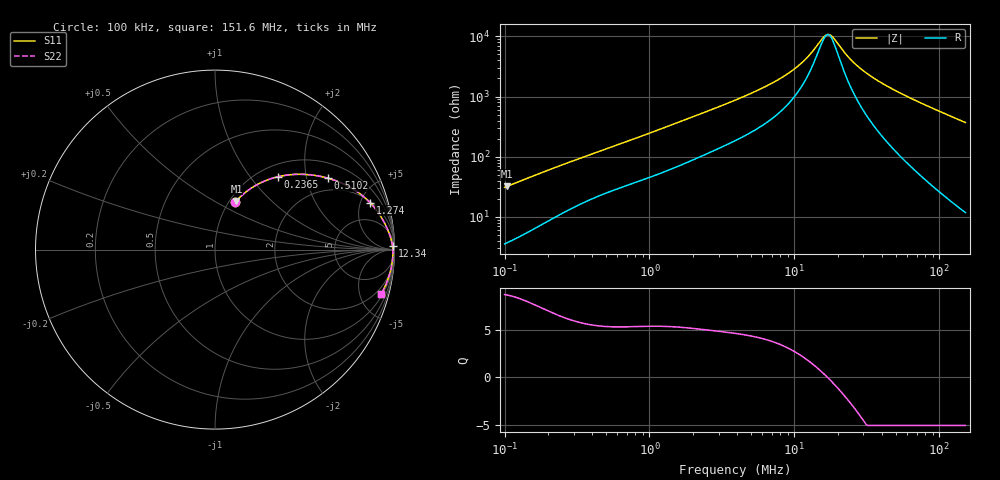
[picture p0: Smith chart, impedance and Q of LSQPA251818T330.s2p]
! LSQPA251818T330  S-PARAMETER MODEL  ( General Type )
! Model Generated by TAIYO YUDEN Corporation (http://www.ty-top.com)
! Version 3.0
! TAIYO YUDEN Control No. 160907NF25SB-FAC
! Copyright(c) 2007 TAIYO YUDEN CO.,LTD. All Rights Reserved.
! Product Description (link to TY-COMPAS)
! https://ds.yuden.co.jp/TYCOMPAS/or/detail?pn=LSQPA251818T330K&u=M
! Products Name : Inductors
! Characteristics :
!  Inductance : 33 uH , SRF(min) : 15 MHz , DC Resistance(max) : 1.95 Ohm
!  Rated Current : Saturation :270 mA , Temp Rise : 320 mA (40 degC)
!  Case Size : 2.5 x 1.8 / 0.098 x 0.071 [mm/inch] , Thickness : 1.8 / 0.071 [mm/inch]
!  (Conditions: Temperature = 25 degC , DC Bias Current/Voltage = 0A / 0V)
! External Node Assignments :
!  1  o---GGG---o  2
! GND o---------o GND
! Frequency Range : 0.1MHz  -  151.640846MHz  [ 402 STEP ]
# MHz S RI R 50
! Freq[MHz].  S11 Real  S11 Imag  S21 Real  S21 Imag  S12 Real  S12 Imag  S22 Real  S22 Imag
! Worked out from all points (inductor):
!   401 points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, 100 kHz to 151.6 MHz, reference 50 ohm
!   read as one part in series: L = 48.6 uH near 103.7 kHz
!   highest Q = 8.6 at 103.7 kHz (marker M1), where L = 49 uH
!   self-resonance near 16.85 MHz
!   S11 on the Smith chart (normalised r, x): 100 kHz: 1.07, +0.62; 236.5 kHz: 1.21, +1.38; 510.2 kHz: 1.51, +2.68; 1.274 MHz: 2.13, +6.03; 12.34 MHz: 45, +79; 151.6 MHz: 1.24, -7.40
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0.1  0.113 0.264  0.887 -0.264  0.887 -0.264  0.113 0.264
0.10373  0.1193 0.2712  0.8807 -0.2712  0.8807 -0.2712  0.1193 0.2712
0.152369  0.2065 0.3453  0.7935 -0.3453  0.7935 -0.3453  0.2065 0.3453
0.236454  0.3494 0.4056  0.6506 -0.4056  0.6506 -0.4056  0.3494 0.4056
0.341025  0.485 0.4195  0.515 -0.4195  0.515 -0.4195  0.485 0.4195
0.51019  0.6283 0.3981  0.3717 -0.3981  0.3717 -0.3981  0.6283 0.3981
1.162983  0.8481 0.2774  0.1519 -0.2774  0.1519 -0.2774  0.8481 0.2774
1.274482  0.8642 0.2614  0.1358 -0.2614  0.1358 -0.2614  0.8642 0.2614
3.894109  0.9645 0.106  0.0355 -0.106  0.0355 -0.106  0.9645 0.106
7.953123  0.9839 0.047  0.0161 -0.047  0.0161 -0.047  0.9839 0.047
10.09053  0.9871 0.0314  0.0129 -0.0314  0.0129 -0.0314  0.9871 0.0314
12.34203  0.989 0.0189  0.011 -0.0189  0.011 -0.0189  0.989 0.0189
13.2799  0.9896 0.0146  0.0104 -0.0146  0.0104 -0.0146  0.9896 0.0146
15.94833  0.9905 0.00371  0.00947 -0.00371  0.00947 -0.00371  0.9905 0.00371
17.47734  0.9909 -0.0017  0.00915 0.0017  0.00915 0.0017  0.9909 -0.0017
18.46424  0.991 -0.00497  0.00901 0.00497  0.00901 0.00497  0.991 -0.00497
23.00149  0.9912 -0.0184  0.00881 0.0184  0.00881 0.0184  0.9912 -0.0184
27.12217  0.9909 -0.029  0.00906 0.029  0.00906 0.029  0.9909 -0.029
33.78694  0.99 -0.0445  0.00997 0.0445  0.00997 0.0445  0.99 -0.0445
45.28783  0.9874 -0.0686  0.0126 0.0686  0.0126 0.0686  0.9874 -0.0686
78.44093  0.9748 -0.1302  0.0252 0.1302  0.0252 0.1302  0.9748 -0.1302
151.6408  0.9252 -0.2475  0.0748 0.2475  0.0748 0.2475  0.9252 -0.2475
